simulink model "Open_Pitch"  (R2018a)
settings: Solver=ode45  StartTime=0.0  StopTime=10  RelTol=1e-3  EnableMultiTasking=on
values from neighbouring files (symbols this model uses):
  Aact = [0, 1; -omg^2, -2*zet*omg]    [init.m]
  Bact = [0; omg^2]    [init.m]
  Cact = [1,0]    [init.m]
  Cza = -0.073    [init.m]
  Czelv = [0.51664,0.51664,0.60478,0.60478,0.06]/100    [init.m]
  d2r = pi/180    (= 0.0174532925199)    [init.m]
  Dact = 0    [init.m]
  Mass = 198.32    [init.m]    (also in lqr_des.m)
  Qbar = 150    [init.m]    (also in lqr_des.m)
  r2d = 180/pi    (= 57.2957795131)    [init.m]    (also in pl.m)
  Sref = 79.069    [init.m]    (also in lqr_des.m)
undefined symbols (not defined in the file or in its folder): Ap, Bp, Cp, Dp, Kmix_qa, Kq

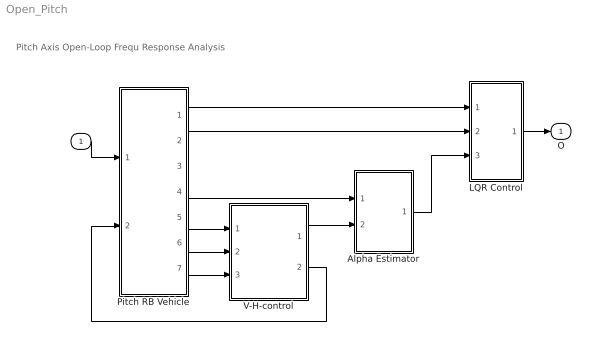
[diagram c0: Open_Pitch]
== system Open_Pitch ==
  note: Pitch Axis Open-Loop Frequ Response Analysis
  I : Inport
  Alpha Estimator : Subsystem
  LQR Control : Subsystem
  Pitch RB Vehicle : Subsystem
  V-H-control : Subsystem
  O : Outport
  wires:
  Pitch RB Vehicle/4("delv ") -> Alpha Estimator/1(delta)
  V-H-control/1(Zdd-com) -> Alpha Estimator/2(Zdd)
  Pitch RB Vehicle/5("Az ") -> V-H-control/1(Az)
  Pitch RB Vehicle/7(Vdot) -> V-H-control/3(Vdot)
  Pitch RB Vehicle/1(thet) -> LQR Control/1(thet)
  Pitch RB Vehicle/2(q) -> LQR Control/2(q)
  Pitch RB Vehicle/6("dH ") -> V-H-control/2(dH)
  V-H-control/2(Throt) -> Pitch RB Vehicle/2(Thro)
  I/1 -> Pitch RB Vehicle/1(delv)
  LQR Control/1(delv) -> O/1
  Alpha Estimator/1(alphat) -> LQR Control/3(alfa)

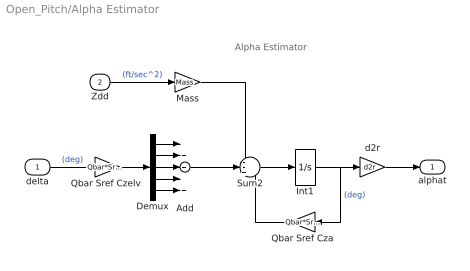
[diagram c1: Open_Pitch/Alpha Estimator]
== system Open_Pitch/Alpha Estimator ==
  note: Alpha Estimator
  delta : Inport
  Zdd : Inport  Port=2
  Add : Sum  Inputs=+++++
  Demux : Demux  Outputs=5
  Int1 : Integrator
  Mass : Gain  Gain=Mass
  Qbar Sref Cza : Gain  Gain=Qbar*Sref*Cza
  "Qbar Sref Czelv " : Gain  Gain=Qbar*Sref*Czelv
  Sum2 : Sum  Inputs=--+
  d2r : Gain  Gain=d2r
  alphat : Outport
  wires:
  Add/1 -> Sum2/2
  Demux/5 -> Add/5
  Demux/4 -> Add/4
  Demux/3 -> Add/3
  Demux/2 -> Add/2
  Demux/1 -> Add/1
  "Qbar Sref Czelv "/1 -> Demux/1
  delta/1 -> "Qbar Sref Czelv "/1  "(deg)"
  Sum2/1 -> Int1/1
  Int1/1 -> d2r/1, Qbar Sref Cza/1  "(deg)"
  Qbar Sref Cza/1 -> Sum2/3
  Zdd/1 -> Mass/1  "(ft/sec^2)"
  Mass/1 -> Sum2/1
  d2r/1 -> alphat/1

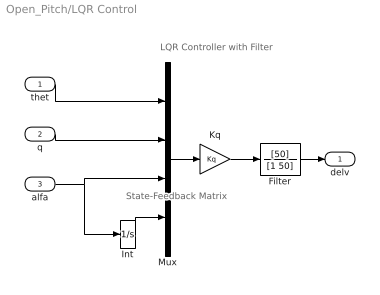
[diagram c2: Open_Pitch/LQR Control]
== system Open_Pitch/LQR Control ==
  note: LQR Controller with Filter
  note: State-Feedback Matrix
  thet : Inport
  q : Inport  Port=2
  alfa : Inport  Port=3
  Filter : TransferFcn  Numerator=[50]  Denominator=[1 50]
  Int : Integrator
  Kq : Gain  Gain=Kq  Multiplication=Matrix(K*u)
  Mux : Mux
  delv : Outport
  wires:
  Kq/1 -> Filter/1
  Mux/1 -> Kq/1
  Int/1 -> Mux/4
  Filter/1 -> delv/1
  q/1 -> Mux/2
  thet/1 -> Mux/1
  alfa/1 -> Mux/3, Int/1

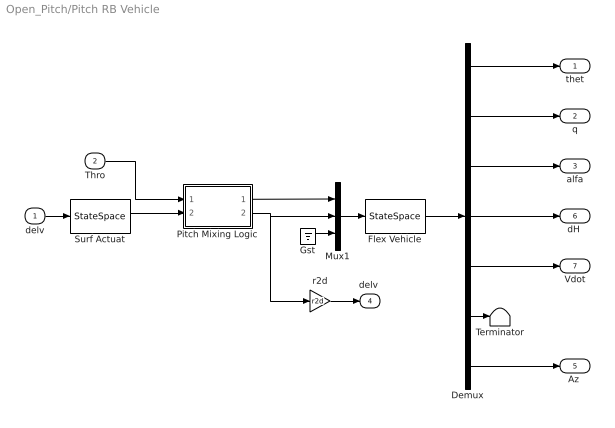
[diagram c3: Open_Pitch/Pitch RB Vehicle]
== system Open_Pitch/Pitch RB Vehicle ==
  delv : Inport
  Thro : Inport  Port=2
  Demux : Demux  Outputs=7
  Flex Vehicle : StateSpace  A=Ap  B=Bp  C=Cp  D=Dp  InitialCondition=0
  Gst : Ground
  Mux1 : Mux  Inputs=[1, 5, 1]
  Pitch Mixing Logic : Subsystem
  Surf Actuat : StateSpace  A=Aact  B=Bact  C=Cact  D=Dact  InitialCondition=0
  Terminator : Terminator
  r2d : Gain  Gain=r2d
  thet : Outport
  q : Outport  Port=2
  alfa : Outport  Port=3
  "delv " : Outport  Port=4
  "Az " : Outport  Port=5
  "dH " : Outport  Port=6
  Vdot : Outport  Port=7
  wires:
  Demux/7 -> "Az "/1
  Demux/3 -> alfa/1
  Demux/2 -> q/1
  Demux/1 -> thet/1
  delv/1 -> Surf Actuat/1
  Mux1/1 -> Flex Vehicle/1
  Flex Vehicle/1 -> Demux/1
  r2d/1 -> "delv "/1
  Thro/1 -> Pitch Mixing Logic/1(Throt)
  Demux/5 -> Vdot/1
  Demux/4 -> "dH "/1
  Gst/1 -> Mux1/3
  Pitch Mixing Logic/2(delta) -> Mux1/2, r2d/1
  Surf Actuat/1 -> Pitch Mixing Logic/2(elev)
  Pitch Mixing Logic/1(Thro) -> Mux1/1
  Demux/6 -> Terminator/1

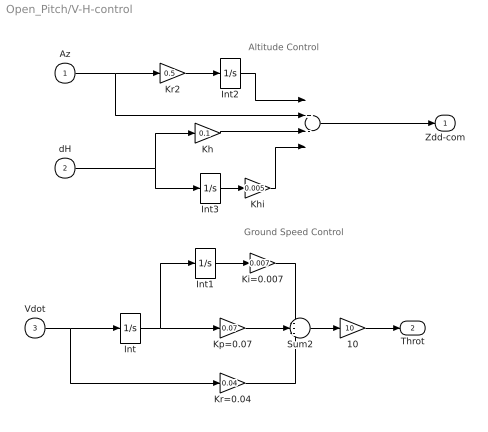
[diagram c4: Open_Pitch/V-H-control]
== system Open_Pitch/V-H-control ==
  note: Ground Speed Control
  note: Altitude Control
  Az : Inport
  dH : Inport  Port=2
  Vdot : Inport  Port=3
  "  " : Sum  Inputs=++--
  10 : Gain  Gain=10
  Int{,1..3} (4 alike) : Integrator
  Kh : Gain  Gain=0.1
  Khi : Gain  Gain=0.005
  Ki=0.007 : Gain  Gain=0.007
  Kp=0.07 : Gain  Gain=0.07
  Kr2 : Gain  Gain=0.5
  Kr=0.04 : Gain  Gain=0.04
  Sum2 : Sum  Inputs=---
  Zdd-com : Outport
  Throt : Outport  Port=2
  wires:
  Khi/1 -> "  "/4
  Int3/1 -> Khi/1
  "  "/1 -> Zdd-com/1
  Az/1 -> "  "/2, Kr2/1
  Int2/1 -> "  "/1
  Kr2/1 -> Int2/1
  Kh/1 -> "  "/3
  dH/1 -> Int3/1, Kh/1
  Int/1 -> Int1/1, Kp=0.07/1
  Int1/1 -> Ki=0.007/1
  Ki=0.007/1 -> Sum2/1
  Kp=0.07/1 -> Sum2/2
  Kr=0.04/1 -> Sum2/3
  Sum2/1 -> 10/1
  Vdot/1 -> Kr=0.04/1, Int/1
  10/1 -> Throt/1

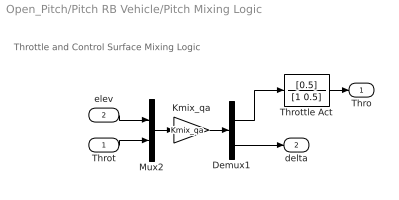
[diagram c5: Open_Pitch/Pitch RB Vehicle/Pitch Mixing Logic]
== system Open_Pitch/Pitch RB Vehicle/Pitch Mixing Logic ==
  note: Throttle and Control Surface Mixing Logic
  Throt : Inport
  elev : Inport  Port=2
  Demux1 : Demux  Outputs=[1, 5]
  Kmix_qa : Gain  Gain=Kmix_qa  Multiplication=Matrix(K*u) (u vector)
  Mux2 : Mux  Inputs=2
  Throttle Act : TransferFcn  Numerator=[0.5]  Denominator=[1 0.5]
  Thro : Outport
  delta : Outport  Port=2
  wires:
  Kmix_qa/1 -> Demux1/1
  Mux2/1 -> Kmix_qa/1
  Demux1/1 -> Throttle Act/1
  Demux1/2 -> delta/1
  elev/1 -> Mux2/1
  Throt/1 -> Mux2/2
  Throttle Act/1 -> Thro/1
